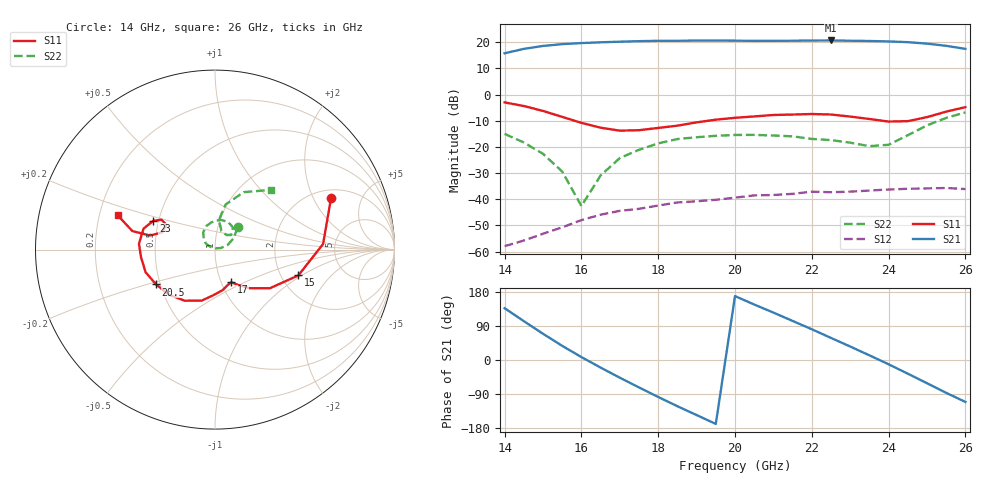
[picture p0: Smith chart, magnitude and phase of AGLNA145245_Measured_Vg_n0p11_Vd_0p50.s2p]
! Filename4Jim: AG10_M047_M4_0307_Vg_n0p11_Vd_0p50_CP3_NF.s2p
! Calibration: TFN_AG02
! Notes: BK
! Row:3, Col:7
! Probes: GSG150
! Prober: TS150
! Date: 2023-12-07 12:27:02
! DC: Vg.V=-0.11262, Vg.I=-5.19342e-07, Vd.V=0.500043, Vd.I=0.0194978
! Keysight Technologies,N5245B,MY58421923,A.15.75.19
! AGMDC-PNAX50 Thu Dec 07 12:27:15 2023
# HZ S DB R 50
!freq (Hz)  S11DB  S11A  S21DB  S21A  S12DB  S12A  S22DB  S22A
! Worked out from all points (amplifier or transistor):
!   25 points, 14 GHz to 26 GHz, reference 50 ohm
!   highest |S21| = 20.7 dB at 22.5 GHz (marker M1)
!   |S21| within 3 dB of that: 14.59 GHz to 25.91 GHz (11.31 GHz wide, 55.9 % of centre)
!   unconditionally stable (mu >= 1): start of sweep to end of sweep
!   at 16 GHz: K = 11.97, MAG = 20.0 dB, |S12| = -48.0 dB
!   at 20 GHz: K = 3.73, MAG = 21.3 dB, |S12| = -39.4 dB
!   at 26 GHz: K = 2.55, MAG = 19.9 dB, |S12| = -36.1 dB
!   lowest NFmin = 1.35 dB at 21 GHz
!   S11 on the Smith chart (normalised r, x): 14 GHz: 2.40, +2.77; 15 GHz: 2.48, -0.94; 17 GHz: 1.12, -0.42; 20.5 GHz: 0.47, -0.22; 23 GHz: 0.47, +0.17; 26 GHz: 0.28, +0.16
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1.4e10  -3.00 24.0  15.75 136.7  -57.93 -13.7  -15.04 44.4
1.45e10  -4.39 3.0  17.45 102.5  -55.78 -49.6  -18.31 31.1
1.5e10  -6.26 -17.2  18.56 69.2  -53.19 -86.7  -22.64 20.2
1.55e10  -8.54 -35.1  19.25 37.4  -50.74 -115.1  -29.43 15.0
1.6e10  -10.82 -48.4  19.65 7.8  -47.97 -136.8  -42.59 73.3
1.65e10  -12.67 -57.4  19.95 -20.1  -45.91 -161.7  -30.92 148.4
1.7e10  -13.81 -63.2  20.18 -46.7  -44.44 173.0  -24.28 146.6
1.75e10  -13.62 -69.4  20.39 -72.4  -43.67 155.6  -21.11 135.0
1.8e10  -12.76 -79.4  20.52 -97.6  -42.41 140.2  -18.65 124.5
1.9e10  -10.65 -104.5  20.61 -145.3  -40.78 102.4  -16.32 97.5
1.95e10  -9.60 -120.6  20.60 -168.7  -40.21 87.0  -15.78 86.8
2e10  -8.89 -135.7  20.58 168.6  -39.41 70.5  -15.44 77.3
2.05e10  -8.37 -149.4  20.50 146.5  -38.53 52.2  -15.42 66.9
2.15e10  -7.65 -174.2  20.55 103.1  -37.94 15.1  -15.98 51.0
2.2e10  -7.43 175.6  20.63 81.1  -37.11 -7.7  -16.97 46.8
2.25e10  -7.64 163.6  20.66 58.3  -37.32 -29.6  -17.40 44.6
2.3e10  -8.42 155.1  20.55 35.6  -37.10 -48.7  -18.39 42.5
2.35e10  -9.34 150.8  20.46 12.3  -36.68 -69.9  -19.73 51.7
2.4e10  -10.33 153.0  20.28 -11.3  -36.29 -92.1  -19.21 71.0
2.5e10  -8.65 167.8  19.44 -61.3  -35.86 -138.5  -11.79 76.9
2.55e10  -6.53 167.4  18.61 -86.6  -35.70 -161.6  -8.94 63.5
2.6e10  -4.83 160.6  17.44 -110.7  -36.12 175.6  -6.84 46.9
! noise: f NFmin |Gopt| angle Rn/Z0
1.4e+10  2.083  0.4394  -52.51  0.5792
1.5e+10  2.049  0.1604  -7.635  0.6163
1.65e+10  1.72  0  90  0.1215
1.8e+10  1.501  0.1893  29.17  0.2101
1.9e+10  1.515  0.1377  123.4  0.425
2.05e+10  1.455  0.1247  121.7  0.3373
2.2e+10  1.526  0  90  0.1053
2.3e+10  1.578  0.1229  157.6  0.2324
2.45e+10  1.602  0  90  0.1115
2.6e+10  2.17  0.03839  54.53  1.755
